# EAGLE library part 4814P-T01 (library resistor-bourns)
BOURNS RESISTOR NETWORK
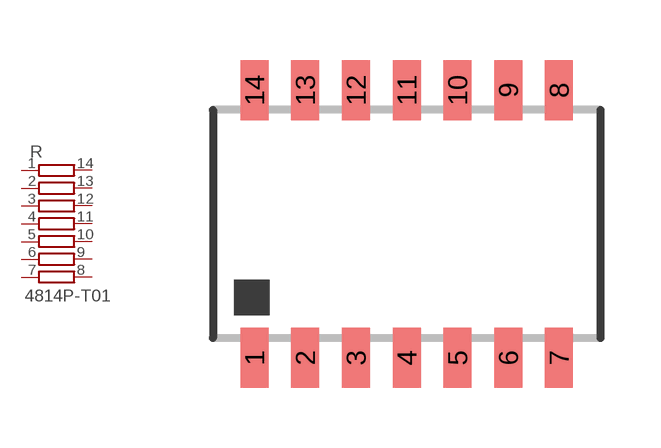
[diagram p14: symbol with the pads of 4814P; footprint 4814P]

Designator prefix R

## 4814P-T01 (MF: BOURNS, INC.; MPN: 4814P-T01-104LF; OC_FARNELL: 9357386; OC_NEWARK: 33K0526)  [4814P]
1  1  pas
2  2  pas
3  3  pas
4  4  pas
5  5  pas
6  6  pas
7  7  pas
8  8  pas
9  9  pas
10  10  pas
11  11  pas
12  12  pas
13  13  pas
14  14  pas

## Footprint 4814P (pad centres in mm)
BOURNS RESISTOR NETWORK
smd 0.7 x 1.5: 1 -3.81,-3.346; 2 -2.54,-3.346; 3 -1.27,-3.346; 4 0,-3.346; 5 1.27,-3.346; 6 2.54,-3.346; 7 3.81,-3.346; 8 3.81,3.346; 9 2.54,3.346; 10 1.27,3.346; 11 0,3.346; 12 -1.27,3.346; 13 -2.54,3.346; 14 -3.81,3.346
